(* 	
	Program Name: 	ACS_MOVE_FORCE
	Purpose:		Copy Force Move Profile to ACS Drive Output Registers
	When Executed:	Primes Output Registers for an Force Move to be executed upon Start Motion command
*)
PROGRAM ACS_MOVE_FORCE
VAR_IN_OUT
	Axis:ACS_DRIVE_TYPE;
END_VAR

VAR_INPUT
	// Position in mm or rotary units
	ProfilePosition		:REAL;
	// Velocity in mm/s or rotary units
	ProfileVelocity		:REAL;
	// Acceleration in mm/s*s or rotary units
	ProfileAcceleration	:REAL;
	//Deceleration in mm/s*s or rotary units
	ProfileDeceleration	:REAL;
	// Force as % Peak motor current
	ProfileForce		:REAL;
END_VAR

VAR
	_moveType:UDINT := ACS_MOTION_TYPES.FORCE;
	// Target Index
	_moveSelect:USINT := 0;
END_VAR

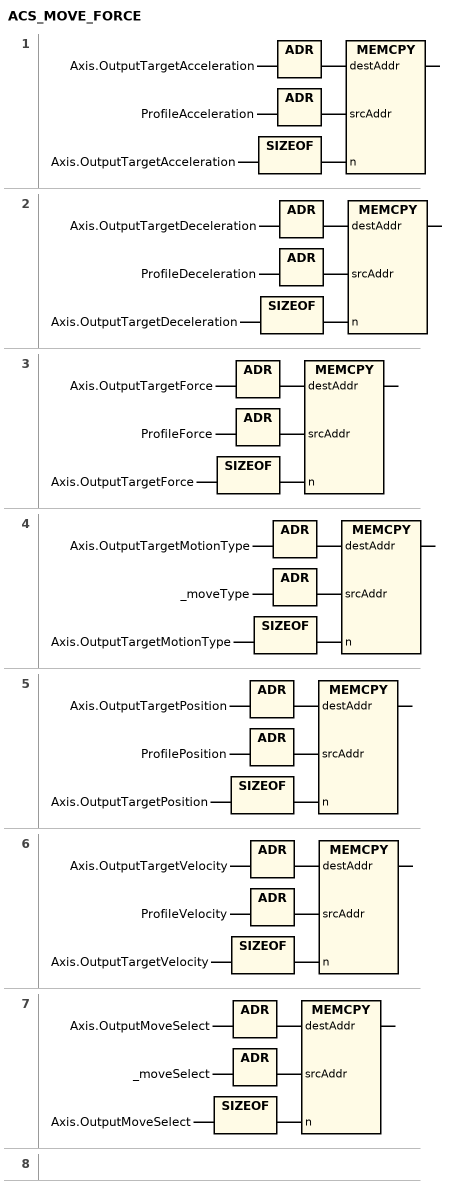
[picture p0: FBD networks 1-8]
// NETWORK 1
MEMCPY(destAddr := ADR(Axis.OutputTargetAcceleration), srcAddr := ADR(ProfileAcceleration), n := SIZEOF(Axis.OutputTargetAcceleration));

// NETWORK 2
MEMCPY(destAddr := ADR(Axis.OutputTargetDeceleration), srcAddr := ADR(ProfileDeceleration), n := SIZEOF(Axis.OutputTargetDeceleration));

// NETWORK 3
MEMCPY(destAddr := ADR(Axis.OutputTargetForce), srcAddr := ADR(ProfileForce), n := SIZEOF(Axis.OutputTargetForce));

// NETWORK 4
MEMCPY(destAddr := ADR(Axis.OutputTargetMotionType), srcAddr := ADR(_moveType), n := SIZEOF(Axis.OutputTargetMotionType));

// NETWORK 5
MEMCPY(destAddr := ADR(Axis.OutputTargetPosition), srcAddr := ADR(ProfilePosition), n := SIZEOF(Axis.OutputTargetPosition));

// NETWORK 6
MEMCPY(destAddr := ADR(Axis.OutputTargetVelocity), srcAddr := ADR(ProfileVelocity), n := SIZEOF(Axis.OutputTargetVelocity));

// NETWORK 7
MEMCPY(destAddr := ADR(Axis.OutputMoveSelect), srcAddr := ADR(_moveSelect), n := SIZEOF(Axis.OutputMoveSelect));

// NETWORK 8

END_PROGRAM
